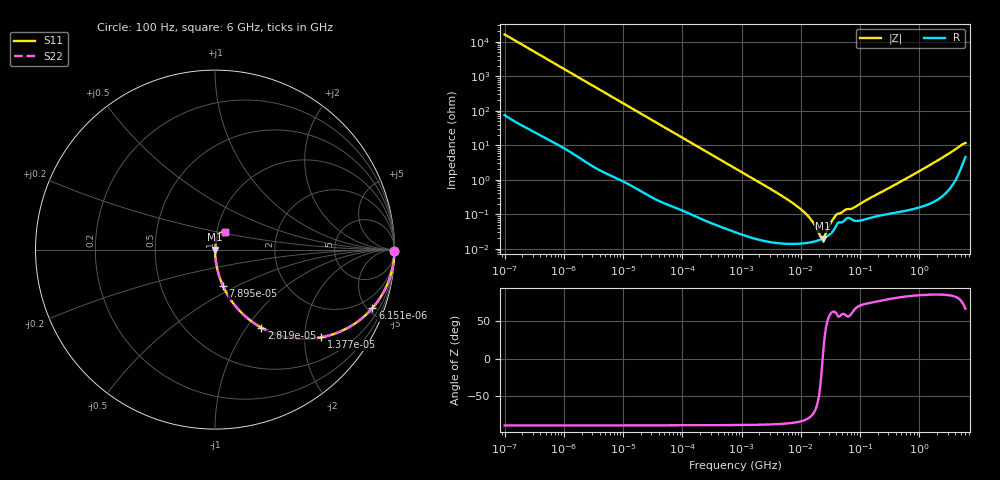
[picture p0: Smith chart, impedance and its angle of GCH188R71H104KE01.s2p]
!Murata Part Number: GCH188R71H104KE01
!These Parameters are Measured in Series Mode Connection
!Data Generated on Jun 19, 2026
!  o--ll--o
!Port1  Port2
!  o------o
!Operation Temp=25[degC], DC Bias Voltage=0[V]
!Freq. Start=100[Hz] Stop=6[GHz] 401[Steps]
# Hz S RI R 50
!Freq.(Hz) S11(Real) S11(Imag) S21(Real) S21(Imag) S12(Real) S12(Imag) S22(Real) S22(Imag)
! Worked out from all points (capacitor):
!   401 points, 100 Hz to 6 GHz, reference 50 ohm
!   read as one part in series: C = 97.3 nF near 109 Hz
!   lowest |Z| = 19.5 mohm at 23.28 MHz (marker M1)
!   series resonance near 23.37 MHz, so ESL is about 480 pH
!   S11 on the Smith chart (normalised r, x): 100 Hz: open; 6.151 kHz: 1.03, -5.37; 13.77 kHz: 1.01, -2.41; 28.19 kHz: 1.01, -1.18; 78.95 kHz: 1.00, -0.42; 6 GHz: 1.09, +0.21
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100  0.9999 -0.00612  6.55e-05 0.00612  6.55e-05 0.00612  0.9999 -0.00612
627  0.9984 -0.0381  0.00164 0.0381  0.00164 0.0381  0.9984 -0.0381
2008  0.9848 -0.1199  0.0152 0.1199  0.0152 0.1199  0.9848 -0.1199
6151  0.8771 -0.3258  0.1229 0.3258  0.1229 0.3258  0.8771 -0.3258
13772  0.5911 -0.4888  0.4089 0.4888  0.4089 0.4888  0.5911 -0.4888
28191  0.259 -0.4353  0.741 0.4353  0.741 0.4353  0.259 -0.4353
40335  0.1468 -0.351  0.8532 0.351  0.8532 0.351  0.1468 -0.351
78952  0.044 -0.2016  0.956 0.2016  0.956 0.2016  0.044 -0.2016
211427  0.00694 -0.0786  0.9931 0.0786  0.9931 0.0786  0.00694 -0.0786
774597  0.000775 -0.0217  0.9992 0.0217  0.9992 0.0217  0.000775 -0.0217
6948629  0.000143 -0.00223  0.9999 0.00223  0.9999 0.00223  0.000143 -0.00223
1.137099e7  0.000145 -0.00115  0.9999 0.00115  0.9999 0.00115  0.000145 -0.00115
1.555665e7  0.000156 -0.000613  0.9998 0.000613  0.9998 0.000613  0.000156 -0.000613
2.128304e7  0.000182 -0.000138  0.9998 0.000138  0.9998 0.000138  0.000182 -0.000138
2.327686e7  0.000195 -6.1e-06  0.9998 6.1e-06  0.9998 6.1e-06  0.000195 -6.1e-06
2.545746e7  0.00021 0.000127  0.9998 -0.000127  0.9998 -0.000127  0.00021 0.000127
3.482834e7  0.000323 0.000628  0.9997 -0.000628  0.9997 -0.000628  0.000323 0.000628
4.165952e7  0.000546 0.000865  0.9995 -0.000865  0.9995 -0.000865  0.000546 0.000865
5.699437e7  0.000718 0.00116  0.9993 -0.00116  0.9993 -0.00116  0.000718 0.00116
7.797396e7  0.000663 0.00138  0.9993 -0.00138  0.9993 -0.00138  0.000663 0.00138
3.124326e8  0.00106 0.00573  0.9989 -0.00573  0.9989 -0.00573  0.00106 0.00573
6e9  0.0533 0.0964  0.9467 -0.0964  0.9467 -0.0964  0.0533 0.0964
